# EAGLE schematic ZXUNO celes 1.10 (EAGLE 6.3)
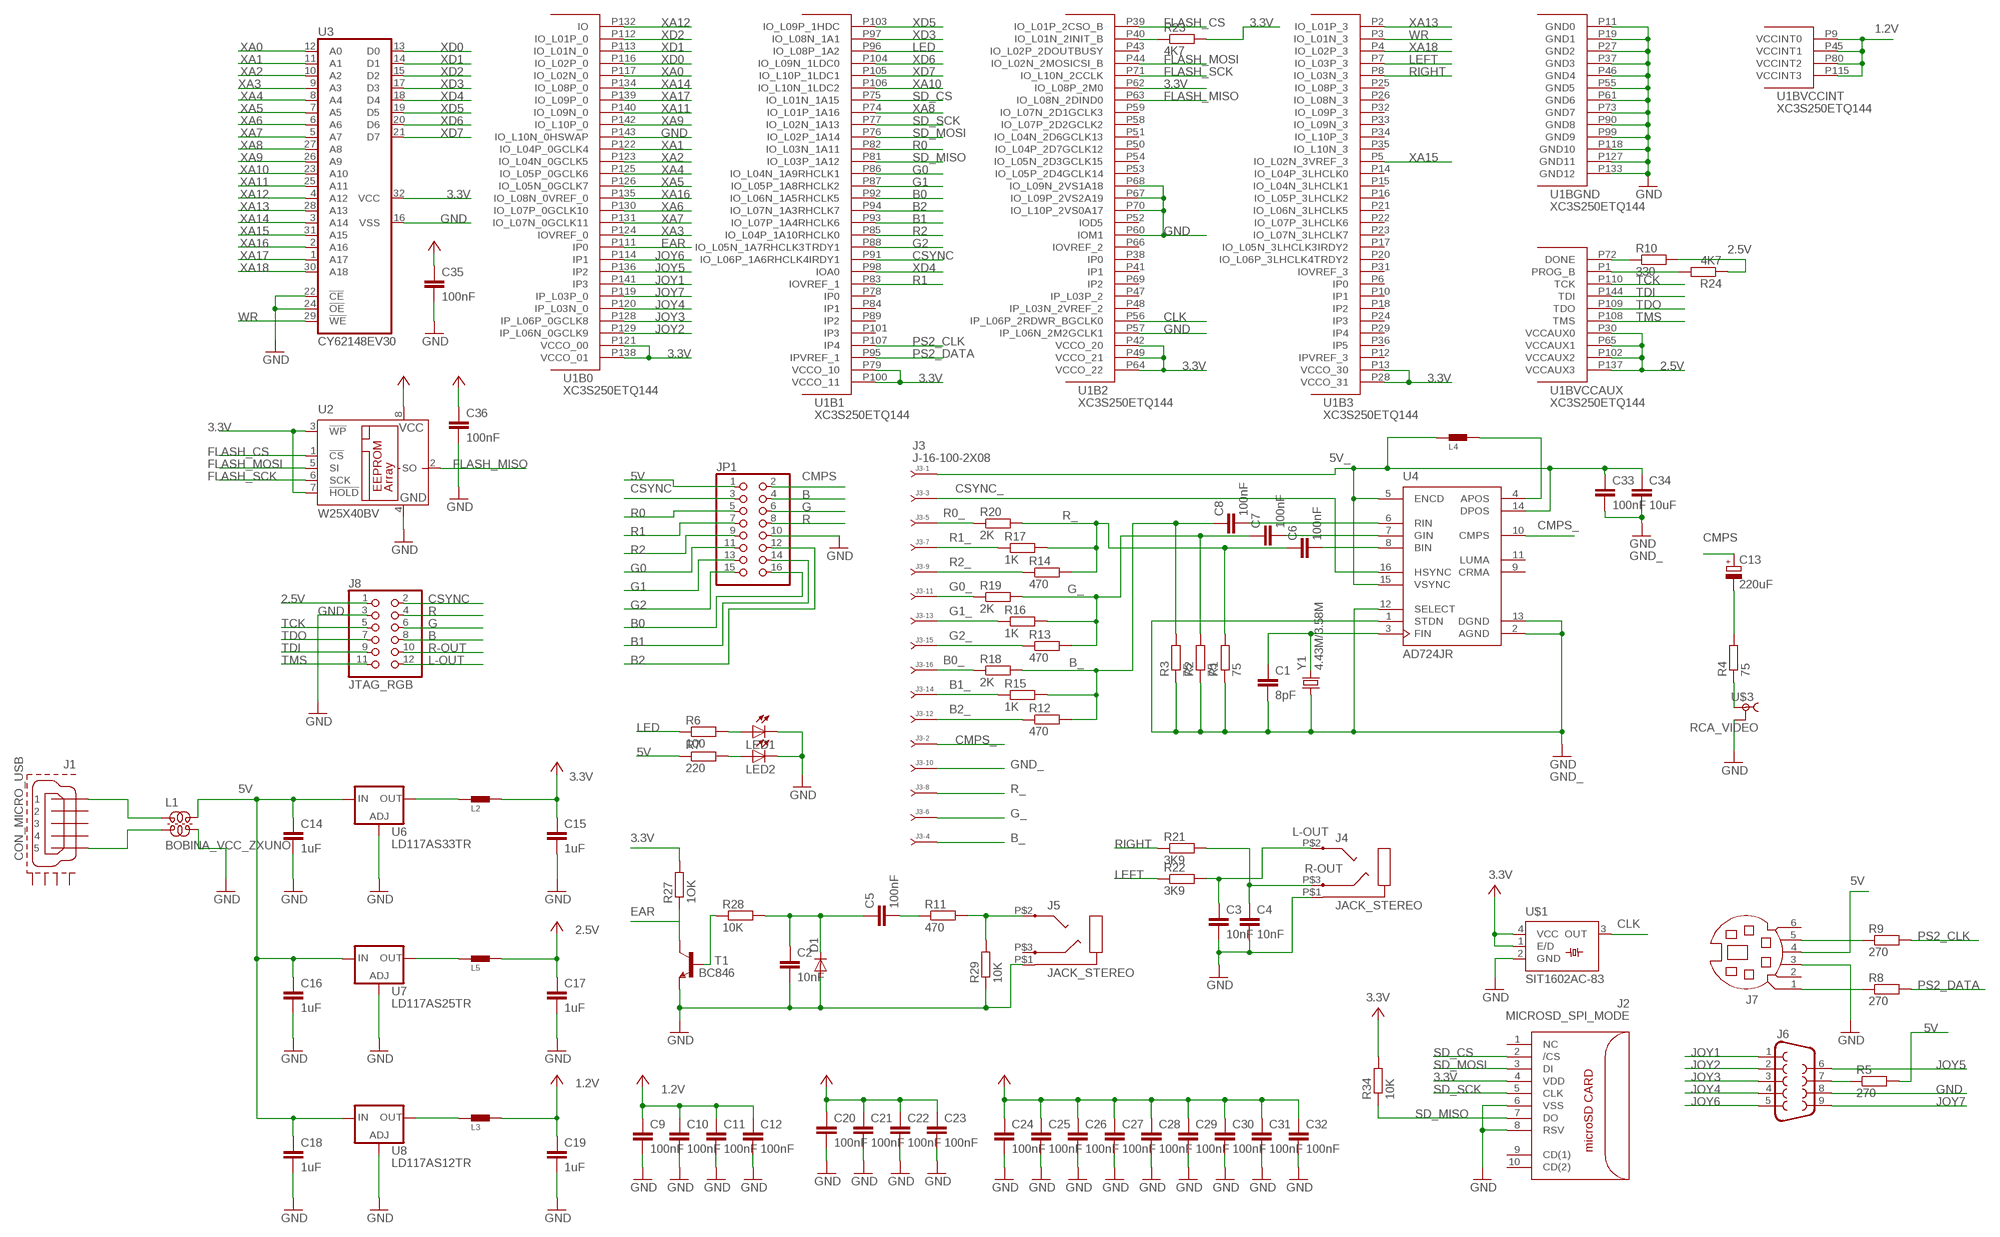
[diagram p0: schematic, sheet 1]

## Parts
C1  8pF  C-EUC0805  [C0805]
C2  10nF  C-EUC0805  [C0805]
C3  10nF  C-EUC0805  [C0805]
C4  10nF  C-EUC0805  [C0805]
C5  100nF  C-EUC0805  [C0805]
C6  100nF  C-EUC0805  [C0805]
C7  100nF  C-EUC0805  [C0805]
C8  100nF  C-EUC0805  [C0805]
C9  100nF  C-EUC0805  [C0805]
C10  100nF  C-EUC0805  [C0805]
C11  100nF  C-EUC0805  [C0805]
C12  100nF  C-EUC0805  [C0805]
C13  220uF  CPOL-EUE5-10.5  [E5-10,5]
C14  1uF  C-EUC0805  [C0805]
C15  1uF  C-EUC0805  [C0805]
C16  1uF  C-EUC0805  [C0805]
C17  1uF  C-EUC0805  [C0805]
C18  1uF  C-EUC0805  [C0805]
C19  1uF  C-EUC0805  [C0805]
C20  100nF  C-EUC0805  [C0805]
C21  100nF  C-EUC0805  [C0805]
C22  100nF  C-EUC0805  [C0805]
C23  100nF  C-EUC0805  [C0805]
C24  100nF  C-EUC0805  [C0805]
C25  100nF  C-EUC0805  [C0805]
C26  100nF  C-EUC0805  [C0805]
C27  100nF  C-EUC0805  [C0805]
C28  100nF  C-EUC0805  [C0805]
C29  100nF  C-EUC0805  [C0805]
C30  100nF  C-EUC0805  [C0805]
C31  100nF  C-EUC0805  [C0805]
C32  100nF  C-EUC0805  [C0805]
C33  100nF  C-EUC0805  [C0805]
C34  10uF  C-EUC0805  [C0805]
C35  100nF  C-EUC0805  [C0805]
C36  100nF  C-EUC0805  [C0805]
D1  DIODE-SOD123  [SOD123]
J1  CON_MICRO_USB  [MICRO_USB]
J2  MICROSD_SPI_MODE  [MICRO_SD_CONNECTOR]
J3  J-16-100-2X08  [DIL-100-2X08]
J4  JACK_STEREO  [STX]
J5  JACK_STEREO  [STX]
J6  F09H  [F09H]
J7  MD06SS  [MDIN06SS]
J8  JTAG_RGB  PINHD-2X6/90  [2X06/90]
JP1  PINHD-2X8  [2X08]
L1  BOBINA_VCC_ZXUNO  [CHOKE_COMM]
L2  FERRITE  [0805]
L3  FERRITE  [0805]
L4  FERRITE  [0805]
L5  FERRITE  [0805]
LED1  LEDCHIPLED_1206  [CHIPLED_1206]
LED2  LEDCHIPLED_1206  [CHIPLED_1206]
R1  75  R-EU_R0805  [R0805]
R2  75  R-EU_R0805  [R0805]
R3  75  R-EU_R0805  [R0805]
R4  75  R-EU_R0805  [R0805]
R5  270  R-EU_R0805  [R0805]
R6  100  R-EU_R0805  [R0805]
R7  220  R-EU_R0805  [R0805]
R8  270  R-EU_R0805  [R0805]
R9  270  R-EU_R0805  [R0805]
R10  330  R-EU_R0805  [R0805]
R11  470  R-EU_R0805  [R0805]
R12  470  R-EU_R0805  [R0805]
R13  470  R-EU_R0805  [R0805]
R14  470  R-EU_R0805  [R0805]
R15  1K  R-EU_R0805  [R0805]
R16  1K  R-EU_R0805  [R0805]
R17  1K  R-EU_R0805  [R0805]
R18  2K  R-EU_R0805  [R0805]
R19  2K  R-EU_R0805  [R0805]
R20  2K  R-EU_R0805  [R0805]
R21  3K9  R-EU_R0805  [R0805]
R22  3K9  R-EU_R0805  [R0805]
R23  4K7  R-EU_R0805  [R0805]
R24  4K7  R-EU_R0805  [R0805]
R27  1OK  R-EU_R0805  [R0805]
R28  10K  R-EU_R0805  [R0805]
R29  10K  R-EU_R0805  [R0805]
R34  10K  R-EU_R0805  [R0805]
T1  BC846  [SOT23]
U1  XC3S250ETQ144  [TQ144]
U2  W25X40BV  25AA080SN  [SO-08]
U3  CY62148EV30  MEMORIAZXUNO  [SOIC32]
U4  AD724JR  [SO16W]
U6  LD117AS33TR  [SOT223]
U7  LD117AS25TR  [SOT223]
U8  LD117AS12TR  [SOT223]
U$1  SIT1602AC-83  [SM77H]
U$3  RCA_VIDEO  [RCA_PACK]
Y1  4.43M/3.58M  CRYSTALHC18U-V  [HC18U-V]

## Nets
1.2V: C9.1 C10.1 C11.1 C12.1 C19.1 L3.2 U1.P9(BVCCINT:VCCINT0) U1.P45(BVCCINT:VCCINT1) U1.P80(BVCCINT:VCCINT2) U1.P115(BVCCINT:VCCINT3) ; supply symbol labelled +3V3
2.5V [alimentacion]: C17.1 C20.1 C21.1 C22.1 C23.1 J8.1 L5.2 R10.2 R24.1 U1.P30(BVCCAUX:VCCAUX0) U1.P65(BVCCAUX:VCCAUX1) U1.P102(BVCCAUX:VCCAUX2) U1.P137(BVCCAUX:VCCAUX3) ; supply symbol labelled +3V3
3.3V [alimentacion]: C15.1 C24.1 C25.1 C26.1 C27.1 C28.1 C29.1 C30.1 C31.1 C32.1 C35.1 C36.1 J2.4(VDD) L2.2 R23.2 R27.2 R34.2 U1.P13(B3:VCCO_30) U1.P28(B3:VCCO_31) U1.P42(B2:VCCO_20) U1.P49(B2:VCCO_21) U1.P62(B2:IO_L08P_2M0) U1.P64(B2:VCCO_22) U1.P79(B1:VCCO_10) U1.P100(B1:VCCO_11) U1.P121(B0:VCCO_00) U1.P138(B0:VCCO_01) U2.3(!WP) U2.7(!HOLD) U2.8(VCC) U3.32(VCC) U$1.1(E/D) U$1.4(VCC) ; supply symbol labelled +3V3
5V [alimentacion]: C14.1 C16.1 C18.1 J7.4 JP1.1 L1.P$4 R5.2 R7.1 U6.3(IN) U7.3(IN) U8.3(IN)
5V_ [alimentacion]: C33.1 C34.1 J3.1 L4.1 U4.5(ENCD) U4.14(DPOS) U4.15(VSYNC)
B: J8.8 JP1.4
B0: JP1.16 U1.P92(B1:IO_L06N_1A5RHCLK5)
B0_: J3.16 R18.1
B1: JP1.14 U1.P93(B1:IO_L07P_1A4RHCLK6)
B1_: J3.14 R15.1
B2: JP1.12 U1.P94(B1:IO_L07N_1A3RHCLK7)
B2_: J3.12 R12.1
B_: C8.1 J3.4 R3.2 R12.2 R15.2 R18.2
CLK: U1.P56(B2:IP_L06P_2RDWR_BGCLK0) U$1.3(OUT)
CMPS: C13.+ JP1.2
CMPS_: J3.2 U4.10(CMPS)
CSYNC: J8.2 JP1.3 U1.P91(B1:IO_L06P_1A6RHCLK4IRDY1)
CSYNC_: J3.3 U4.16(HSYNC)
EAR: R27.1 T1.3(C) U1.P111(B0:IP0)
FLASH_CS: U1.P39(B2:IO_L01P_2CSO_B) U2.1(!CS)
FLASH_MISO: U1.P63(B2:IO_L08N_2DIND0) U2.2(SO)
FLASH_MOSI: U1.P44(B2:IO_L02N_2MOSICSI_B) U2.5(SI)
FLASH_SCK: U1.P71(B2:IO_L10N_2CCLK) U2.6(SCK)
G: J8.6 JP1.6
G0: JP1.11 U1.P86(B1:IO_L04N_1A9RHCLK1)
G0_: J3.11 R19.1
G1: JP1.13 U1.P87(B1:IO_L05P_1A8RHCLK2)
G1_: J3.13 R16.1
G2: JP1.15 U1.P88(B1:IO_L05N_1A7RHCLK3TRDY1)
G2_: J3.15 R13.1
G_: C7.1 J3.6 R2.2 R13.2 R16.2 R19.2
GND [alimentacion]: C2.2 C3.2 C4.2 C9.2 C10.2 C11.2 C12.2 C14.2 C15.2 C16.2 C17.2 C18.2 C19.2 C20.2 C21.2 C22.2 C23.2 C24.2 C25.2 C26.2 C27.2 C28.2 C29.2 C30.2 C31.2 C32.2 C35.2 C36.2 D1.A J2.6(VSS) J2.8(RSV) J4.P$1 J5.P$1 J6.8 J7.3 J8.3 JP1.10 L1.P$3 LED1.C LED2.C R29.1 T1.2(E) U1.P11(BGND:GND0) U1.P19(BGND:GND1) U1.P27(BGND:GND2) U1.P37(BGND:GND3) U1.P46(BGND:GND4) U1.P55(BGND:GND5) U1.P57(B2:IP_L06N_2M2GCLK1) U1.P60(B2:IOM1) U1.P61(BGND:GND6) U1.P67(B2:IO_L09P_2VS2A19) U1.P68(B2:IO_L09N_2VS1A18) U1.P70(B2:IO_L10P_2VS0A17) U1.P73(BGND:GND7) U1.P90(BGND:GND8) U1.P99(BGND:GND9) U1.P118(BGND:GND10) U1.P127(BGND:GND11) U1.P133(BGND:GND12) U1.P143(B0:IO_L10N_0HSWAP) U2.4(GND) U3.16(VSS) U3.22(!CE) U3.24(!OE) U6.1(ADJ) U7.1(ADJ) U8.1(ADJ) U$1.2(GND) U$3.1
GND_ [alimentacion]: C1.2 C33.2 C34.2 J3.10 R1.1 R2.1 R3.1 U4.1(STDN) U4.2(AGND) U4.12(SELECT) U4.13(DGND) Y1.1 ; supply symbol labelled GND
JOY1: J6.1 U1.P141(B0:IP3)
JOY2: J6.2 U1.P129(B0:IP_L06N_0GCLK9)
JOY3: J6.3 U1.P128(B0:IP_L06P_0GCLK8)
JOY4: J6.4 U1.P120(B0:IP_L03N_0)
JOY5: J6.6 U1.P136(B0:IP2)
JOY6: J6.5 U1.P114(B0:IP1)
JOY7: J6.9 U1.P119(B0:IP_L03P_0)
L-OUT: C3.1 J4.P$2 J8.12 R22.2
LED: R6.1 U1.P96(B1:IO_L08P_1A2)
LEFT: R22.1 U1.P7(B3:IO_L03P_3)
N$1: C8.2 U4.6(RIN)
N$2: C7.2 U4.7(GIN)
N$3: C6.2 U4.8(BIN)
N$5: LED1.A R6.2
N$6: C1.1 U4.3(FIN) Y1.2
N$8: LED2.A R7.2
N$9: C13.- R4.2
N$10: R4.1 U$3.2 U$3.2@1
N$11: R28.1 T1.1(B)
N$12: C2.1 C5.1 D1.C R28.2
N$13: C5.2 R11.1
N$14: J5.P$2 R11.2 R29.2
N$15: R24.2 U1.P1(BVCCAUX:PROG_B)
N$16: R10.1 U1.P72(BVCCAUX:DONE)
N$17: R23.1 U1.P40(B2:IO_L01N_2INIT_B)
N$18: J7.1 R8.1
N$19: J7.5 R9.1
N$20: J6.7 R5.1
N$21 [alimentacion]: L2.1 U6.2(OUT) U6.4(OUT)
N$22 [alimentacion]: L5.1 U7.2(OUT) U7.4(OUT)
N$23 [alimentacion]: L3.1 U8.2(OUT) U8.4(OUT)
N$24: L4.2 U4.4(APOS)
N$25 [alimentacion]: J1.1 L1.P$1
N$26 [alimentacion]: J1.5 L1.P$2
PS2_CLK: R9.2 U1.P107(B1:IP4)
PS2_DATA: R8.2 U1.P95(B1:IPVREF_1)
R: J8.4 JP1.8
R0: JP1.5 U1.P82(B1:IO_L03N_1A11)
R0_: J3.5 R20.1
R1: JP1.7 U1.P83(B1:IOVREF_1)
R1_: J3.7 R17.1
R2: JP1.9 U1.P85(B1:IO_L04P_1A10RHCLK0)
R2_: J3.9 R14.1
R-OUT: C4.1 J4.P$3 J8.10 R21.2
R_: C6.1 J3.8 R1.2 R14.2 R17.2 R20.2
RIGHT: R21.1 U1.P8(B3:IO_L03N_3)
SD_CS: J2.2(/CS) U1.P75(B1:IO_L01N_1A15)
SD_MISO: J2.7(DO) R34.1 U1.P81(B1:IO_L03P_1A12)
SD_MOSI: J2.3(DI) U1.P76(B1:IO_L02P_1A14)
SD_SCK: J2.5(CLK) U1.P77(B1:IO_L02N_1A13)
TCK: J8.5 U1.P110(BVCCAUX:TCK)
TDI: J8.9 U1.P144(BVCCAUX:TDI)
TDO: J8.7 U1.P109(BVCCAUX:TDO)
TMS: J8.11 U1.P108(BVCCAUX:TMS)
WR: U1.P3(B3:IO_L01N_3) U3.29(!WE)
XA0: U1.P117(B0:IO_L02N_0) U3.12(A0)
XA1: U1.P122(B0:IO_L04P_0GCLK4) U3.11(A1)
XA2: U1.P123(B0:IO_L04N_0GCLK5) U3.10(A2)
XA3: U1.P124(B0:IOVREF_0) U3.9(A3)
XA4: U1.P125(B0:IO_L05P_0GCLK6) U3.8(A4)
XA5: U1.P126(B0:IO_L05N_0GCLK7) U3.7(A5)
XA6: U1.P130(B0:IO_L07P_0GCLK10) U3.6(A6)
XA7: U1.P131(B0:IO_L07N_0GCLK11) U3.5(A7)
XA8: U1.P74(B1:IO_L01P_1A16) U3.27(A8)
XA9: U1.P142(B0:IO_L10P_0) U3.26(A9)
XA10: U1.P106(B1:IO_L10N_1LDC2) U3.23(A10)
XA11: U1.P140(B0:IO_L09N_0) U3.25(A11)
XA12: U1.P132(B0:IO) U3.4(A12)
XA13: U1.P2(B3:IO_L01P_3) U3.28(A13)
XA14: U1.P134(B0:IO_L08P_0) U3.3(A14)
XA15: U1.P5(B3:IO_L02N_3VREF_3) U3.31(A15)
XA16: U1.P135(B0:IO_L08N_0VREF_0) U3.2(A16)
XA17: U1.P139(B0:IO_L09P_0) U3.1(A17)
XA18: U1.P4(B3:IO_L02P_3) U3.30(A18)
XD0: U1.P116(B0:IO_L02P_0) U3.13(D0)
XD1: U1.P113(B0:IO_L01N_0) U3.14(D1)
XD2: U1.P112(B0:IO_L01P_0) U3.15(D2)
XD3: U1.P97(B1:IO_L08N_1A1) U3.17(D3)
XD4: U1.P98(B1:IOA0) U3.18(D4)
XD5: U1.P103(B1:IO_L09P_1HDC) U3.19(D5)
XD6: U1.P104(B1:IO_L09N_1LDC0) U3.20(D6)
XD7: U1.P105(B1:IO_L10P_1LDC1) U3.21(D7)
Unconnected: J1.2 J1.3 J1.4 J1.P$1(GND1) J1.P$2(GND2) J1.P$3(GND3) J1.P$4(GND4) J2.1(NC) J2.9(CD(1)) J2.10(CD(2)) J5.P$3 J7.2 J7.6 U1.P6(B3:IP0) U1.P10(B3:IP1) U1.P12(B3:IPVREF_3) U1.P14(B3:IO_L04P_3LHCLK0) U1.P15(B3:IO_L04N_3LHCLK1) U1.P16(B3:IO_L05P_3LHCLK2) U1.P17(B3:IO_L05N_3LHCLK3IRDY2) U1.P18(B3:IP2) U1.P20(B3:IO_L06P_3LHCLK4TRDY2) U1.P21(B3:IO_L06N_3LHCLK5) U1.P22(B3:IO_L07P_3LHCLK6) U1.P23(B3:IO_L07N_3LHCLK7) U1.P24(B3:IP3) U1.P25(B3:IO_L08P_3) U1.P26(B3:IO_L08N_3) U1.P29(B3:IP4) U1.P31(B3:IOVREF_3) U1.P32(B3:IO_L09P_3) U1.P33(B3:IO_L09N_3) U1.P34(B3:IO_L10P_3) U1.P35(B3:IO_L10N_3) U1.P36(B3:IP5) U1.P38(B2:IP0) U1.P41(B2:IP1) U1.P43(B2:IO_L02P_2DOUTBUSY) U1.P47(B2:IP_L03P_2) U1.P48(B2:IP_L03N_2VREF_2) U1.P50(B2:IO_L04P_2D7GCLK12) U1.P51(B2:IO_L04N_2D6GCLK13) U1.P52(B2:IOD5) U1.P53(B2:IO_L05P_2D4GCLK14) U1.P54(B2:IO_L05N_2D3GCLK15) U1.P58(B2:IO_L07P_2D2GCLK2) U1.P59(B2:IO_L07N_2D1GCLK3) U1.P66(B2:IOVREF_2) U1.P69(B2:IP2) U1.P78(B1:IP0) U1.P84(B1:IP1) U1.P89(B1:IP2) U1.P101(B1:IP3) U4.9(CRMA) U4.11(LUMA)

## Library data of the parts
C1-C12 C14-C36 = rcl:C-EU: CAPACITOR, European symbol
C13 = rcl:CPOL-EU: POLARIZED CAPACITOR, European symbol
D1 = diode:DIODE-: DIODE
J1 = ZXUNO:CON_MICRO_USB
J2 = con-molex-microsd:MICROSD_SPI_MODE: MOLEX - 49225-0821 - CONNECTEUR MICRO SD PUSH/PUSH REV Fabricant: MOLEX Code commande Farnell: 1366700 Référence fabricant: 49225-0821
J3 = con-headers-jp:J-16-: HEADER JACK PINS
J4 J5 = ZXUNO:JACK_STEREO
J6 = con-subd:F09: SUB-D; OC_FARNELL: unknown; OC_NEWARK: unknown
J7 = con-yamaichi:MD06SS: YAMAICHI CONNECTOR; OC_FARNELL: unknown; OC_NEWARK: unknown
J8 = pinhead:PINHD-2X6: PIN HEADER
JP1 = pinhead:PINHD-2X8: PIN HEADER
L1 = ZXUNO:BOBINA_VCC_ZXUNO
L2-L5 = Murata AWJLEagleLib:FERRITE: Ferrite bead
LED1 LED2 = led:LED: LED
R1-R24 R27-R29 R34 = rcl:R-EU_: RESISTOR, European symbol
T1 = transistor:BC846: NPN TRANSISTOR
U1 = xilinx_spartan3_virtex4_and_5:XC3S250ETQ144: Xilinx FPGA
U2 = microchip:25*: Serial EEPROM 4K/ 8K , SPI bus; MF: MICROCHIP; MPN: 25AA080/SN; OC_FARNELL: 1816072; OC_NEWARK: 92C7351
U3 = ZXUNO:MEMORIAZXUNO
U4 = vga2tv:AD724
U6-U8 = v-reg:LD117A?*: Low drop fixed and adjustable positive voltage regulators 1 A Source: http://www.st.com/stonline/products/literature/ds/7194/ld1117axx.pdf
U$1 = ZXUNO:SIT1602AC-83
U$3 = ZXUNO:RCA_VIDEO
Y1 = crystal:CRYSTAL: CRYSTAL; OC_FARNELL: unknown; OC_NEWARK: unknown

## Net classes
1 alimentacion: width 0.203 mm, drill 0.203 mm, clearance 0.203 mm

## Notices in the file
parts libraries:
con-headers-jp: Copyright (C) 2008, Bob Starr
